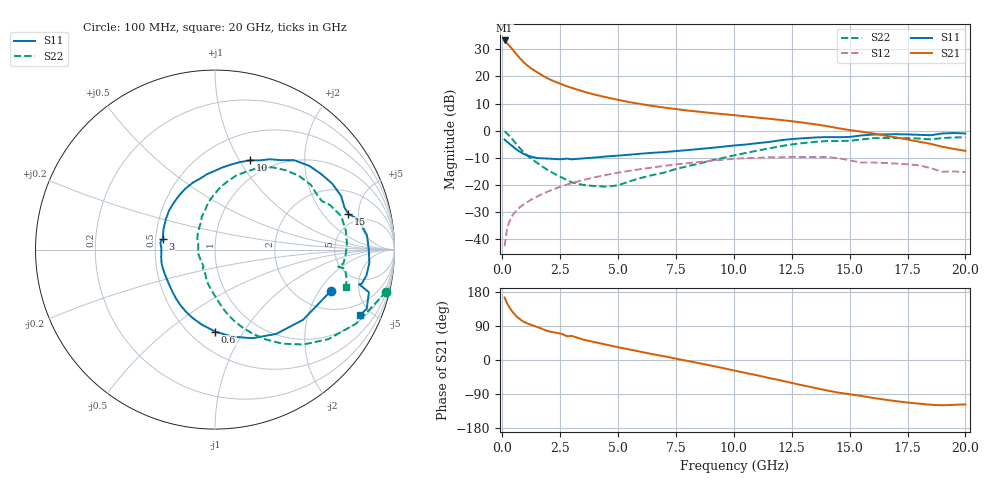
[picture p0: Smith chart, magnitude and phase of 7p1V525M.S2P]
! Infineon Technologies  Discrete & RF Semiconductors
! bfp620
! VCE =  1.5 V,  IC =  25 mA
! Common Emitter S-Parameters:  Sep 2002
# GHz  S  MA  R  50
!  f  S11  S21  S12  S22
! GHz  MAG  ANG  MAG  ANG  MAG  ANG  MAG  ANG
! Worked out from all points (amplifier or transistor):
!   59 points, 100 MHz to 20 GHz, reference 50 ohm
!   highest |S21| = 33.2 dB at 100 MHz (marker M1)
!   |S21| within 3 dB of that: start of sweep to 413.1 MHz
!   unconditionally stable (mu >= 1): 3.221 GHz to 9.883 GHz; 17.16 GHz to end of sweep
!   at 1 GHz: K = 0.73, MSG = 25.7 dB, |S12| = -26.7 dB
!   at 5.5 GHz: K = 1.04, MAG = 11.5 dB, |S12| = -14.8 dB
!   at 20 GHz: K = 1.32, MAG = 0.5 dB, |S12| = -15.2 dB
!   S11 on the Smith chart (normalised r, x): 100 MHz: 3.00, -2.59; 600 MHz: 0.66, -0.76; 3 GHz: 0.55, +0.07; 10 GHz: 0.80, +1.11; 15 GHz: 3.86, +3.75; 20 GHz: 1.25, -4.30
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0.1  0.6868 -19.4  45.85 164.7  0.0075 84.5  0.9827 -13.8
0.2  0.6276 -38.5  41.02 150.6  0.015 73.7  0.8888 -27.6
0.3  0.5806 -54.0  36.87 139.5  0.021 68.6  0.8048 -38.3
0.4  0.5358 -67.2  32.96 130.5  0.0259 65.1  0.723 -47.0
0.5  0.4937 -79.0  29.29 122.8  0.0301 62.5  0.6446 -54.4
0.6  0.4567 -89.8  25.97 116.3  0.0337 60.6  0.5729 -60.7
0.7  0.4258 -99.6  23.09 110.7  0.0371 59.2  0.5099 -66.2
0.9  0.3803 -115.8  18.65 101.9  0.0433 57.6  0.4115 -74.9
1.2  0.3382 -133.1  14.54 93.7  0.0523 56.5  0.3177 -83.4
1.6  0.3129 -150.8  11.27 85.0  0.0645 55.0  0.2395 -92.8
2  0.3068 -166.0  9.021 75.8  0.0769 52.9  0.1851 -103.5
2.8  0.307 172.6  6.554 62.6  0.1021 47.5  0.1233 -123.9
3  0.2975 168.1  6.149 63.7  0.1083 46.0  0.1122 -124.8
3.5  0.3097 157.8  5.268 53.7  0.1241 41.8  0.1003 -141.6
5  0.3478 131.1  3.696 33.7  0.1689 28.2  0.099 160.2
7  0.4043 101.8  2.659 9.7  0.2252 9.3  0.1699 117.5
10  0.5342 68.7  1.937 -27.5  0.3042 -23.4  0.3508 84.8
10.5  0.5558 63.4  1.838 -34.2  0.312 -29.9  0.3872 79.5
13.5  0.7502 29.2  1.314 -73.6  0.3281 -65.7  0.6224 41.4
15  0.7685 15.0  1.026 -90.3  0.2848 -86.8  0.6534 24.5
17  0.863 -4.9  0.755 -108.6  0.2482 -97.3  0.736 2.9
20  0.8873 -24.3  0.425 -117.2  0.1736 -107.5  0.7561 -15.8
